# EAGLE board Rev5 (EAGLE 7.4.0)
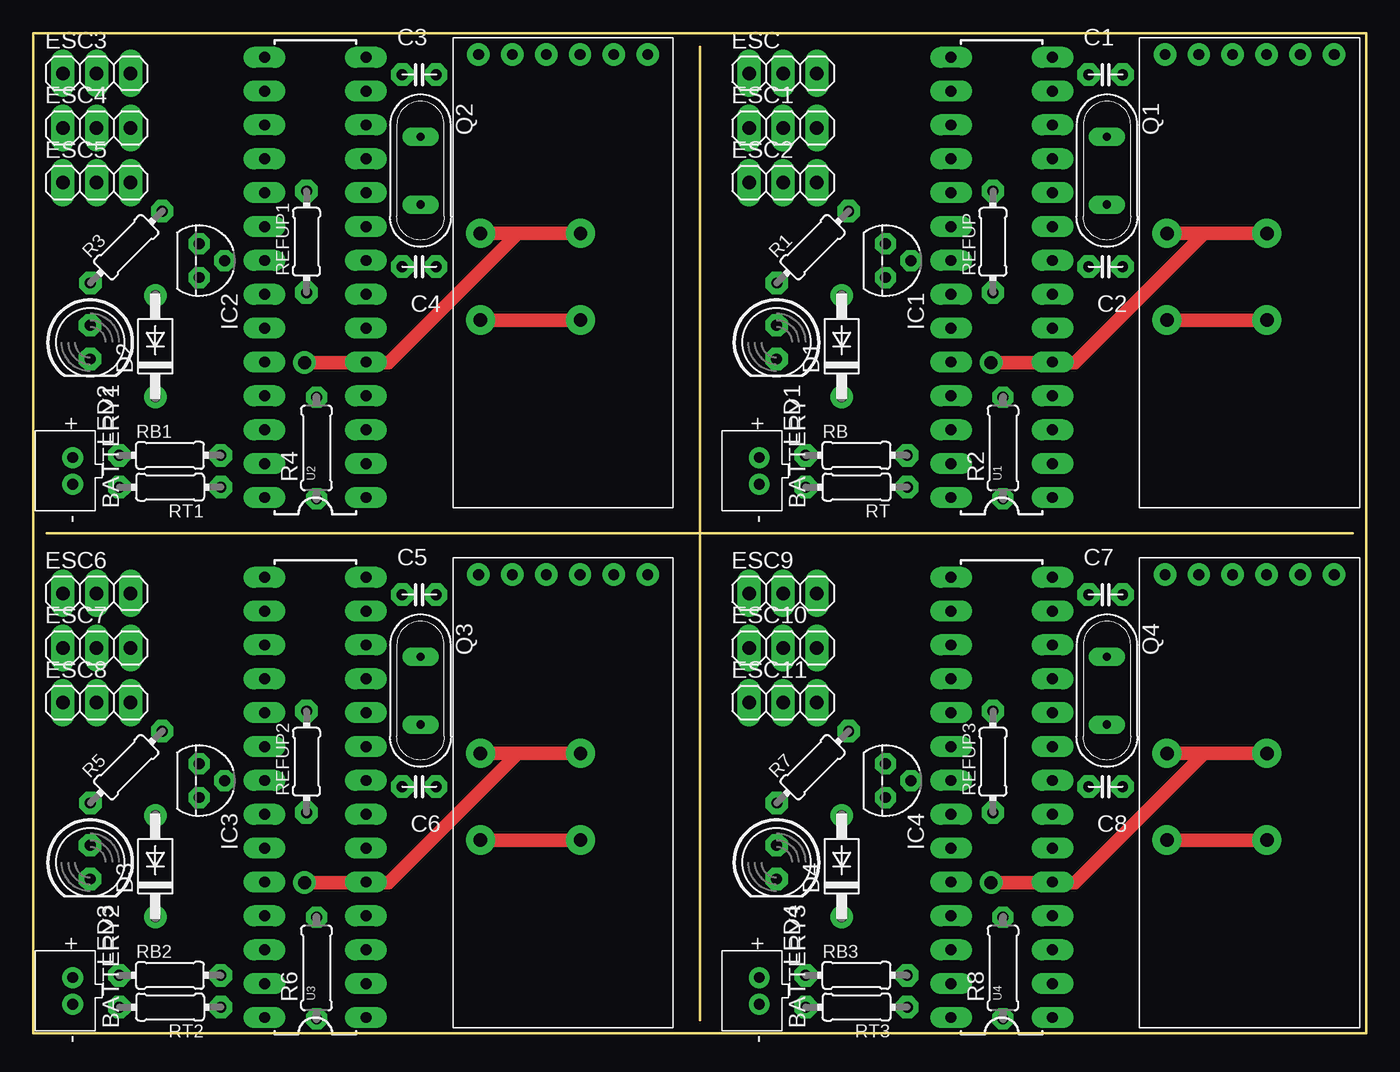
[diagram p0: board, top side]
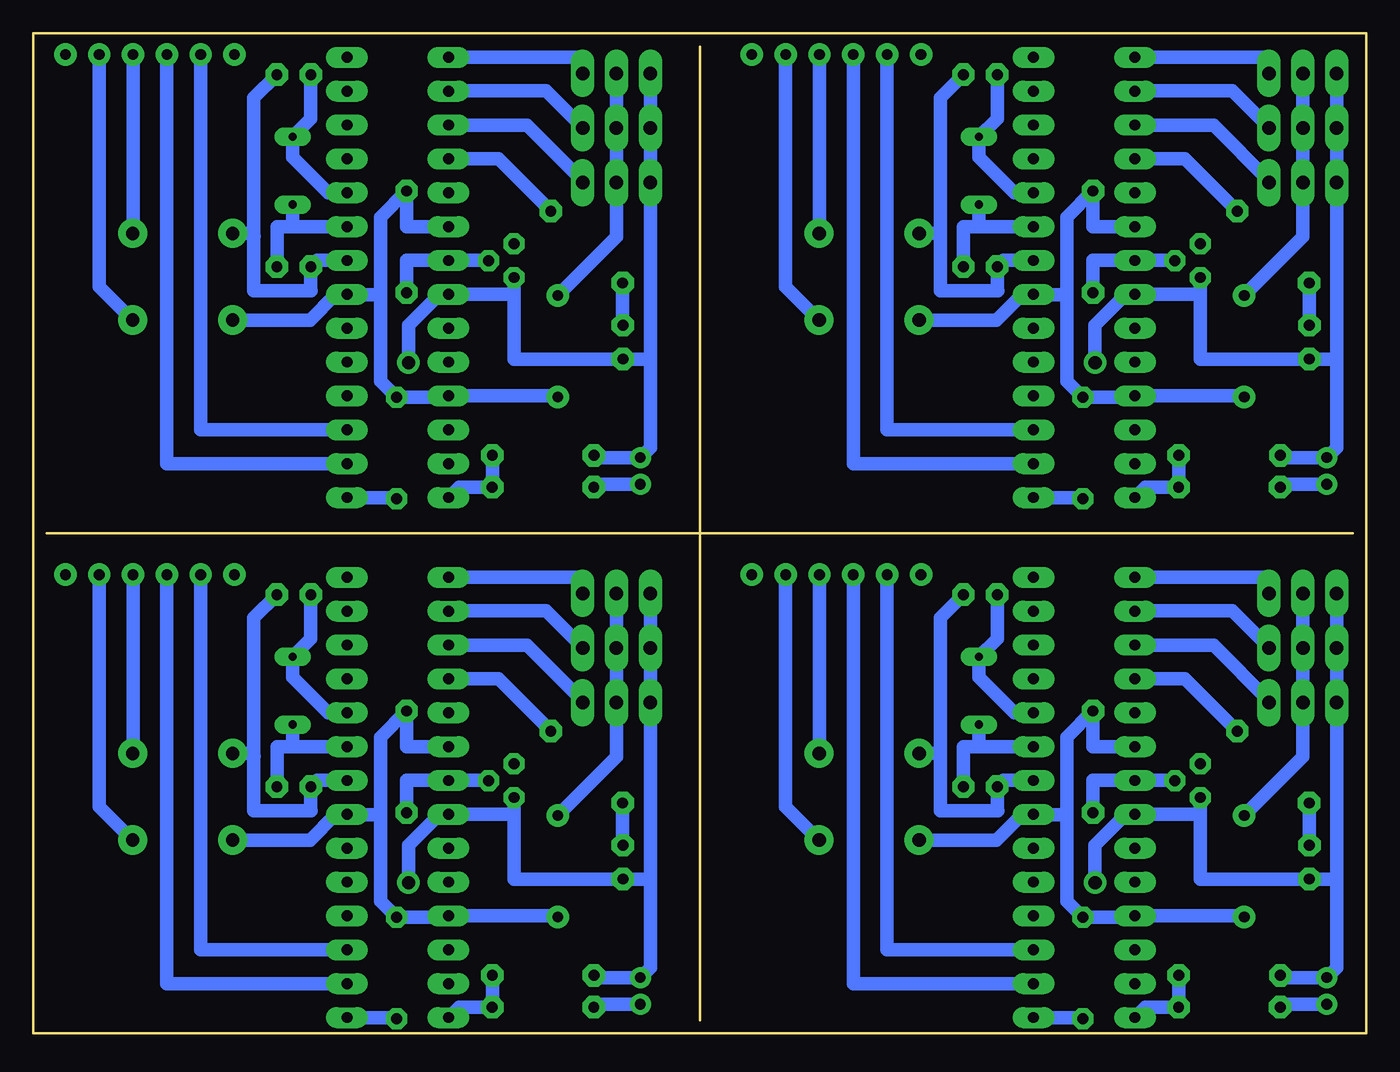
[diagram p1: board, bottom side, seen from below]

Size 100 x 75 mm. Coordinates in mm from the lower left corner, seen from the top.
Outline: 0,0 50,0 100,0 100,37.5 100,75 50,75 0,75 0,37.5 0,0
Copper layers (1*16): Top 0.035mm / dielectric 1.5mm / Bottom 0.035mm
Design rules "default *": minimum track width 10mil, minimum drill 24mil, track to track 15mil, track to pad 15mil, pad to pad 15mil, via to via 15mil, smd to smd 8mil, copper to edge 40mil, drill to drill 8mil, minimum pad ring 15mil, minimum via ring 8mil, stop-mask expansion 4mil, vias tented up to drill 0mil, thermal gap 10mil
Milling: 2 lines

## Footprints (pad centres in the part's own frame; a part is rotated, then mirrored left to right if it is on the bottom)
JST-PH-2-THM = drill 0.8 pad 1.422: 1 1,0; 2 -1,0
C2.5-4 = drill 0.813 pad 1.676 octagon: 1 -1.27,0; 2 1.27,0
DO41-10 = drill 0.8 pad 1.676: A 2.54,0; C -5.08,0
1X03 = drill 1.016 long: 1 -2.54,0; 2 0,0; 3 2.54,0
TO92 = drill 0.813 octagon: 1 -1.27,0; 2 0,1.905; 3 1.27,0
LED5MM = drill 0.813 pad 1.676 octagon: A -1.27,0; K 1.27,0
QS = drill 0.61 long: 1 -2.54,0; 2 2.54,0
0204/7 = drill 0.813 pad 1.676 octagon: 1 -3.81,0; 2 3.81,0
0207/7 = drill 0.813 octagon: 1 -3.81,0; 2 3.81,0
DIL28-3 = drill 0.813 long: 1 -16.51,-3.81; 2 -13.97,-3.81; 3 -11.43,-3.81; 4 -8.89,-3.81; 5 -6.35,-3.81; 6 -3.81,-3.81; 7 -1.27,-3.81; 8 1.27,-3.81; 9 3.81,-3.81; 10 6.35,-3.81; 11 8.89,-3.81; 12 11.43,-3.81; 13 13.97,-3.81; 14 16.51,-3.81; 15 16.51,3.81; 16 13.97,3.81; 17 11.43,3.81; 18 8.89,3.81; 19 6.35,3.81; 20 3.81,3.81; 21 1.27,3.81; 22 -1.27,3.81; 23 -3.81,3.81; 24 -6.35,3.81; 25 -8.89,3.81; 26 -11.43,3.81; 27 -13.97,3.81; 28 -16.51,3.81
HC06 = drill 0.8 pad 1.676: EN -6.35,0; GND -1.27,0; RX 3.81,0; STATE 6.35,0; TX 1.27,0; VCC -3.81,0

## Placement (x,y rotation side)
BATTERY  [JST-PH-2-THM]  54.46,42.18 90 top
BATTERY1  [JST-PH-2-THM]  2.96,42.18 90 top
BATTERY2  [JST-PH-2-THM]  2.96,3.18 90 top
BATTERY3  [JST-PH-2-THM]  54.46,3.18 90 top
C1  [C2.5-4]  80.45,71.9 0 top
C2  [C2.5-4]  80.45,57.5 180 top
C3  [C2.5-4]  28.95,71.9 0 top
C4  [C2.5-4]  28.95,57.5 180 top
C5  [C2.5-4]  28.95,32.9 0 top
C6  [C2.5-4]  28.95,18.5 180 top
C7  [C2.5-4]  80.45,32.9 0 top
C8  [C2.5-4]  80.45,18.5 180 top
D1  1N4933  [DO41-10]  60.65,52.8 90 top
D2  1N4933  [DO41-10]  9.15,52.8 90 top
D3  1N4933  [DO41-10]  9.15,13.8 90 top
D4  1N4933  [DO41-10]  60.65,13.8 90 top
ESC  [1X03]  56.25,72 0 top
ESC1  [1X03]  56.25,67.9 0 top
ESC2  [1X03]  56.25,63.8 0 top
ESC3  [1X03]  4.75,72 0 top
ESC4  [1X03]  4.75,67.9 0 top
ESC5  [1X03]  4.75,63.8 0 top
ESC6  [1X03]  4.75,33 0 top
ESC7  [1X03]  4.75,28.9 0 top
ESC8  [1X03]  4.75,24.8 0 top
ESC9  [1X03]  56.25,33 0 top
ESC10  [1X03]  56.25,28.9 0 top
ESC11  [1X03]  56.25,24.8 0 top
IC1  LM336LP  [TO92]  63.94,57.95 270 top
IC2  LM336LP  [TO92]  12.44,57.95 270 top
IC3  LM336LP  [TO92]  12.44,18.95 270 top
IC4  LM336LP  [TO92]  63.94,18.95 270 top
LED1  [LED5MM]  55.76,51.84 270 top
LED2  [LED5MM]  4.26,51.84 270 top
LED3  [LED5MM]  4.26,12.84 270 top
LED4  [LED5MM]  55.76,12.84 270 top
Q1  [QS]  80.55,64.7 270 top
Q2  [QS]  29.05,64.7 270 top
Q3  [QS]  29.05,25.7 270 top
Q4  [QS]  80.55,25.7 270 top
R1  270  [0204/7]  58.48,58.97 45 top
R2  10000  [0207/7]  72.75,43.9 90 top
R3  270  [0204/7]  6.98,58.97 45 top
R4  10000  [0207/7]  21.25,43.9 90 top
R5  270  [0204/7]  6.98,19.97 45 top
R6  10000  [0207/7]  21.25,4.9 90 top
R7  270  [0204/7]  58.48,19.97 45 top
R8  10000  [0207/7]  72.75,4.9 90 top
RB  20000  [0204/7]  61.75,43.35 0 top
RB1  20000  [0204/7]  10.25,43.35 0 top
RB2  20000  [0204/7]  10.25,4.35 0 top
RB3  20000  [0204/7]  61.75,4.35 0 top
REFUP  3300  [0204/7]  72,59.37 90 top
REFUP1  3300  [0204/7]  20.5,59.37 90 top
REFUP2  3300  [0204/7]  20.5,20.37 90 top
REFUP3  3300  [0204/7]  72,20.37 90 top
RT  220000  [0204/7]  61.76,40.96 180 top
RT1  220000  [0204/7]  10.26,40.96 180 top
RT2  220000  [0204/7]  10.26,1.96 180 top
RT3  220000  [0204/7]  61.76,1.96 180 top
U1  ATMEGA328P_PDIP  [DIL28-3]  72.66,56.7 90 top
U2  ATMEGA328P_PDIP  [DIL28-3]  21.16,56.7 90 top
U3  ATMEGA328P_PDIP  [DIL28-3]  21.16,17.7 90 top
U4  ATMEGA328P_PDIP  [DIL28-3]  72.66,17.7 90 top
U$1  HC06  [HC06]  91.25,73.4 180 top
U$2  HC06  [HC06]  39.75,73.4 180 top
U$3  HC06  [HC06]  39.75,34.4 180 top
U$4  HC06  [HC06]  91.25,34.4 180 top

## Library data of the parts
BATTERY BATTERY1-BATTERY3 LED1-LED4 R1 R3 R5 R7 RB RB1-RB3 REFUP REFUP1-REFUP3 RT RT1-RT3 = adafruit
C1-C8 = capacitor-wima
D1-D4 = diode
ESC ESC1-ESC11 = pinhead
IC1-IC4 = VLADLIBRARY
Q1-Q4 = special
R2 R4 R6 R8 = resistor
U1-U4 = SparkFun-DigitalIC
U$1-U$4 = ccs

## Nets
BUTTON: ESC2.3 U1.17
BUTTON1: ESC5.3 U2.17
BUTTON2: ESC8.3 U3.17
BUTTON3: ESC11.3 U4.17
ESC: ESC.3 U1.15
ESC1: ESC3.3 U2.15
ESC2: ESC6.3 U3.15
ESC3: ESC9.3 U4.15
GND: BATTERY.1 C1.2 C2.2 ESC1.1 ESC2.1 ESC.1 IC1.3 LED1.K RB.1 U1.8 U1.22 U$1.GND
GND1: BATTERY1.1 C3.2 C4.2 ESC3.1 ESC4.1 ESC5.1 IC2.3 LED2.K RB1.1 U2.8 U2.22 U$2.GND
GND2: BATTERY2.1 C5.2 C6.2 ESC6.1 ESC7.1 ESC8.1 IC3.3 LED3.K RB2.1 U3.8 U3.22 U$3.GND
GND3: BATTERY3.1 C7.2 C8.2 ESC9.1 ESC10.1 ESC11.1 IC4.3 LED4.K RB3.1 U4.8 U4.22 U$4.GND
LED: R1.2 U1.18
LED1: R3.2 U2.18
LED2: R5.2 U3.18
LED3: R7.2 U4.18
N$1: BATTERY1.2 RT1.2
N$2: LED1.A R1.1
N$3: C1.1 Q1.1 U1.10
N$4: BATTERY.2 RT.2
N$5: C2.1 Q1.2 U1.9
N$6: LED2.A R3.1
N$7: R2.1 U1.1
N$8: C3.1 Q2.1 U2.10
N$9: C4.1 Q2.2 U2.9
N$10: D1.A ESC1.2 ESC2.2 ESC.2
N$11: R4.1 U2.1
N$12: D2.A ESC3.2 ESC4.2 ESC5.2
N$13: BATTERY2.2 RT2.2
N$14: LED3.A R5.1
N$15: C5.1 Q3.1 U3.10
N$16: C6.1 Q3.2 U3.9
N$17: R6.1 U3.1
N$18: D3.A ESC6.2 ESC7.2 ESC8.2
N$19: BATTERY3.2 RT3.2
N$20: LED4.A R7.1
N$21: C7.1 Q4.1 U4.10
N$22: C8.1 Q4.2 U4.9
N$23: R8.1 U4.1
N$24: D4.A ESC9.2 ESC10.2 ESC11.2
RX: U1.2 U$1.TX
RX1: U2.2 U$2.TX
RX2: U3.2 U$3.TX
RX3: U4.2 U$4.TX
STEER: ESC1.3 U1.16
STEER1: ESC4.3 U2.16
STEER2: ESC7.3 U3.16
STEER3: ESC10.3 U4.16
TX: U1.3 U$1.RX
TX1: U2.3 U$2.RX
TX2: U3.3 U$3.RX
TX3: U4.3 U$4.RX
VCC: D1.C R2.2 REFUP.2 U1.7 U1.20 U1.25 U$1.VCC
VCC1: D2.C R4.2 REFUP1.2 U2.7 U2.20 U2.25 U$2.VCC
VCC2: D3.C R6.2 REFUP2.2 U3.7 U3.20 U3.25 U$3.VCC
VCC3: D4.C R8.2 REFUP3.2 U4.7 U4.20 U4.25 U$4.VCC
VOLTMETER: RB.2 RT.1 U1.28
VOLTMETER1: RB1.2 RT1.1 U2.28
VOLTMETER2: RB2.2 RT2.1 U3.28
VOLTMETER3: RB3.2 RT3.1 U4.28
VREF: IC1.2 REFUP.1 U1.21
VREF1: IC2.2 REFUP1.1 U2.21
VREF2: IC3.2 REFUP2.1 U3.21
VREF3: IC4.2 REFUP3.1 U4.21

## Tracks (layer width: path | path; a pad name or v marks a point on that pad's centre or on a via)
BUTTON
  Bottom 1.016: ESC2.3 58.79,63.94 62.95,68.1 68.82,68.1 U1.17
BUTTON1
  Bottom 1.016: ESC5.3 7.29,63.94 11.45,68.1 17.32,68.1 U2.17
BUTTON2
  Bottom 1.016: ESC8.3 7.29,24.94 11.45,29.1 17.32,29.1 U3.17
BUTTON3
  Bottom 1.016: ESC11.3 58.79,24.94 62.95,29.1 68.82,29.1 U4.17
ESC
  Bottom 1.016: ESC.3 58.79,73.21 U1.15
ESC1
  Bottom 1.016: ESC3.3 7.29,73.21 U2.15
ESC2
  Bottom 1.016: ESC6.3 7.29,34.21 U3.15
ESC3
  Bottom 1.016: ESC9.3 58.79,34.21 U4.15
GND  (via drill 1 pad 1.68, 1 pad 2.18)
  Top 1.016: v92.55,60 87.85,60 | 87.85,60 v85.05,60 | v71.85,50.3 78.15,50.3 87.85,60
  Bottom 1.016: 53.71,50.57 LED1.K 63.94,50.57 IC1.3 63.94,55.43 U1.22 69.52,55.43 71.85,53.1 v71.85,50.3 | 53.71,50.57 ESC2.1 ESC1.1 ESC.1 | RB.1 57.77,43.18 BATTERY.1 53.71,43.93 53.71,50.57 | U1.8 78.71,57.97 C2.2 79.18,55.73 79.15,55.7 83.45,55.7 83.45,59.8 | C1.2 83.45,70.17 83.45,59.8 | U$1.GND 92.52,60.03 v92.55,60 | v85.05,60 83.65,60 83.45,59.8
GND1  (via drill 1 pad 1.68, 1 pad 2.18)
  Top 1.016: v41.05,60 36.35,60 | 36.35,60 v33.55,60 | v20.35,50.3 26.65,50.3 36.35,60
  Bottom 1.016: 2.21,50.57 LED2.K 12.44,50.57 IC2.3 12.44,55.43 U2.22 18.02,55.43 20.35,53.1 v20.35,50.3 | 2.21,50.57 ESC5.1 ESC4.1 ESC3.1 | RB1.1 6.27,43.18 BATTERY1.1 2.21,43.93 2.21,50.57 | U2.8 27.21,57.97 C4.2 27.68,55.73 27.65,55.7 31.95,55.7 31.95,59.8 | C3.2 31.95,70.17 31.95,59.8 | U$2.GND 41.02,60.03 v41.05,60 | v33.55,60 32.15,60 31.95,59.8
GND2  (via drill 1 pad 1.68, 1 pad 2.18)
  Top 1.016: v41.05,21 36.35,21 | 36.35,21 v33.55,21 | v20.35,11.3 26.65,11.3 36.35,21
  Bottom 1.016: 2.21,11.57 LED3.K 12.44,11.57 IC3.3 12.44,16.43 U3.22 18.02,16.43 20.35,14.1 v20.35,11.3 | 2.21,11.57 ESC8.1 ESC7.1 ESC6.1 | RB2.1 6.27,4.18 BATTERY2.1 2.21,4.93 2.21,11.57 | U3.8 27.21,18.97 C6.2 27.68,16.73 27.65,16.7 31.95,16.7 31.95,20.8 | C5.2 31.95,31.17 31.95,20.8 | U$3.GND 41.02,21.03 v41.05,21 | v33.55,21 32.15,21 31.95,20.8
GND3  (via drill 1 pad 1.68, 1 pad 2.18)
  Top 1.016: v92.55,21 87.85,21 | 87.85,21 v85.05,21 | v71.85,11.3 78.15,11.3 87.85,21
  Bottom 1.016: 53.71,11.57 LED4.K 63.94,11.57 IC4.3 63.94,16.43 U4.22 69.52,16.43 71.85,14.1 v71.85,11.3 | 53.71,11.57 ESC11.1 ESC10.1 ESC9.1 | RB3.1 57.77,4.18 BATTERY3.1 53.71,4.93 53.71,11.57 | U4.8 78.71,18.97 C8.2 79.18,16.73 79.15,16.7 83.45,16.7 83.45,20.8 | C7.2 83.45,31.17 83.45,20.8 | U$4.GND 92.52,21.03 v92.55,21 | v85.05,21 83.65,21 83.45,20.8
LED
  Bottom 1.016: R1.2 65.09,65.59 U1.18
LED1
  Bottom 1.016: R3.2 13.59,65.59 U2.18
LED2
  Bottom 1.016: R5.2 13.59,26.59 U3.18
LED3
  Bottom 1.016: R7.2 65.09,26.59 U4.18
N$1
  Bottom 1.016: RT1.2 6.23,41.18 BATTERY1.2
N$2
  Bottom 1.016: LED1.A 55.78,53.11 R1.1
N$3
  Bottom 1.016: U1.10 77.9,63.05 80.55,65.7 Q1.1 79.18,68.61 C1.1
N$4
  Bottom 1.016: RT.2 57.73,41.18 BATTERY.2
N$5
  Bottom 1.016: Q1.2 80.55,60.51 | 80.55,60.51 U1.9 | C2.1 81.72,60.51 80.55,60.51
N$6
  Bottom 1.016: LED2.A 4.28,53.11 R3.1
N$7
  Bottom 1.016: R2.1 72.85,40.19 U1.1
N$8
  Bottom 1.016: U2.10 26.4,63.05 29.05,65.7 Q2.1 27.68,68.61 C3.1
N$9
  Bottom 1.016: Q2.2 29.05,60.51 | 29.05,60.51 U2.9 | C4.1 30.22,60.51 29.05,60.51
N$10
  Bottom 1.016: ESC.2 ESC1.2 ESC2.2 56.25,59.74 D1.A | ESC.2 56.25,72.8 56.35,72.7 56.35,72.1 | 56.35,72.1 56.35,71.5 | ESC.2 56.35,72.1
N$11
  Bottom 1.016: R4.1 21.35,40.19 U2.1
N$12
  Bottom 1.016: ESC3.2 ESC4.2 ESC5.2 4.75,59.74 D2.A | ESC3.2 4.75,72.8 4.85,72.7 4.85,72.1 | 4.85,72.1 4.85,71.5 | ESC3.2 4.85,72.1
N$13
  Bottom 1.016: RT2.2 6.23,2.18 BATTERY2.2
N$14
  Bottom 1.016: LED3.A 4.28,14.11 R5.1
N$15
  Bottom 1.016: U3.10 26.4,24.05 29.05,26.7 Q3.1 27.68,29.61 C5.1
N$16
  Bottom 1.016: Q3.2 29.05,21.51 | 29.05,21.51 U3.9 | C6.1 30.22,21.51 29.05,21.51
N$17
  Bottom 1.016: R6.1 21.35,1.19 U3.1
N$18
  Bottom 1.016: ESC6.2 ESC7.2 ESC8.2 4.75,20.74 D3.A | ESC6.2 4.75,33.8 4.85,33.7 4.85,33.1 | 4.85,33.1 4.85,32.5 | ESC6.2 4.85,33.1
N$19
  Bottom 1.016: RT3.2 57.73,2.18 BATTERY3.2
N$20
  Bottom 1.016: LED4.A 55.78,14.11 R7.1
N$21
  Bottom 1.016: U4.10 77.9,24.05 80.55,26.7 Q4.1 79.18,29.61 C7.1
N$22
  Bottom 1.016: Q4.2 80.55,21.51 | 80.55,21.51 U4.9 | C8.1 81.72,21.51 80.55,21.51
N$23
  Bottom 1.016: R8.1 72.85,1.19 U4.1
N$24
  Bottom 1.016: ESC9.2 ESC10.2 ESC11.2 56.25,20.74 D4.A | ESC9.2 56.25,33.8 56.35,33.7 56.35,33.1 | 56.35,33.1 56.35,32.5 | ESC9.2 56.35,33.1
RX
  Bottom 1.016: U$1.TX 89.98,42.73 U1.2
RX1
  Bottom 1.016: U$2.TX 38.48,42.73 U2.2
RX2
  Bottom 1.016: U$3.TX 38.48,3.73 U3.2
RX3
  Bottom 1.016: U$4.TX 89.98,3.73 U4.2
STEER
  Bottom 1.016: ESC1.3 58.79,67.94 61.55,70.7 68.81,70.7 U1.16
STEER1
  Bottom 1.016: ESC4.3 7.29,67.94 10.05,70.7 17.31,70.7 U2.16
STEER2
  Bottom 1.016: ESC7.3 7.29,28.94 10.05,31.7 17.31,31.7 U3.16
STEER3
  Bottom 1.016: ESC10.3 58.79,28.94 61.55,31.7 68.81,31.7 U4.16
TX
  Bottom 1.016: U$1.RX 87.44,45.27 U1.3
TX1
  Bottom 1.016: U$2.RX 35.94,45.27 U2.3
TX2
  Bottom 1.016: U$3.RX 35.94,6.27 U3.3
TX3
  Bottom 1.016: U$4.RX 87.44,6.27 U4.3
VCC  (via drill 1 pad 2.18)
  Top 1.016: v92.55,53.5 v85.05,53.5
  Bottom 1.016: U1.20 72,60.51 REFUP.2 73.95,61.22 73.95,55.4 | 73.95,55.4 76.44,55.4 U1.7 76.49,55.4 77.35,55.4 79.25,53.5 v85.05,53.5 | 73.95,55.4 73.95,48.91 R2.2 68.94,47.71 U1.25 60.74,47.81 D1.C | U$1.VCC 95.06,56.01 v92.55,53.5
VCC1  (via drill 1 pad 2.18)
  Top 1.016: v41.05,53.5 v33.55,53.5
  Bottom 1.016: U2.20 20.5,60.51 REFUP1.2 22.45,61.22 22.45,55.4 | 22.45,55.4 24.94,55.4 U2.7 24.99,55.4 25.85,55.4 27.75,53.5 v33.55,53.5 | 22.45,55.4 22.45,48.91 R4.2 17.44,47.71 U2.25 9.24,47.81 D2.C | U$2.VCC 43.56,56.01 v41.05,53.5
VCC2  (via drill 1 pad 2.18)
  Top 1.016: v41.05,14.5 v33.55,14.5
  Bottom 1.016: U3.20 20.5,21.51 REFUP2.2 22.45,22.22 22.45,16.4 | 22.45,16.4 24.94,16.4 U3.7 24.99,16.4 25.85,16.4 27.75,14.5 v33.55,14.5 | 22.45,16.4 22.45,9.91 R6.2 17.44,8.71 U3.25 9.24,8.81 D3.C | U$3.VCC 43.56,17.01 v41.05,14.5
VCC3  (via drill 1 pad 2.18)
  Top 1.016: v92.55,14.5 v85.05,14.5
  Bottom 1.016: U4.20 72,21.51 REFUP3.2 73.95,22.22 73.95,16.4 | 73.95,16.4 76.44,16.4 U4.7 76.49,16.4 77.35,16.4 79.25,14.5 v85.05,14.5 | 73.95,16.4 73.95,9.91 R8.2 68.94,8.71 U4.25 60.74,8.81 D4.C | U$4.VCC 95.06,17.01 v92.55,14.5
VOLTMETER
  Bottom 1.016: U1.28 68.07,40.96 RT.1 65.56,40.97 RB.2
VOLTMETER1
  Bottom 1.016: U2.28 16.57,40.96 RT1.1 14.06,40.97 RB1.2
VOLTMETER2
  Bottom 1.016: U3.28 16.57,1.96 RT2.1 14.06,1.97 RB2.2
VOLTMETER3
  Bottom 1.016: U4.28 68.07,1.96 RT3.1 65.56,1.97 RB3.2
VREF
  Bottom 1.016: IC1.2 65.86,57.97 U1.21 72,57.97 REFUP.1
VREF1
  Bottom 1.016: IC2.2 14.36,57.97 U2.21 20.5,57.97 REFUP1.1
VREF2
  Bottom 1.016: IC3.2 14.36,18.97 U3.21 20.5,18.97 REFUP2.1
VREF3
  Bottom 1.016: IC4.2 65.86,18.97 U4.21 72,18.97 REFUP3.1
